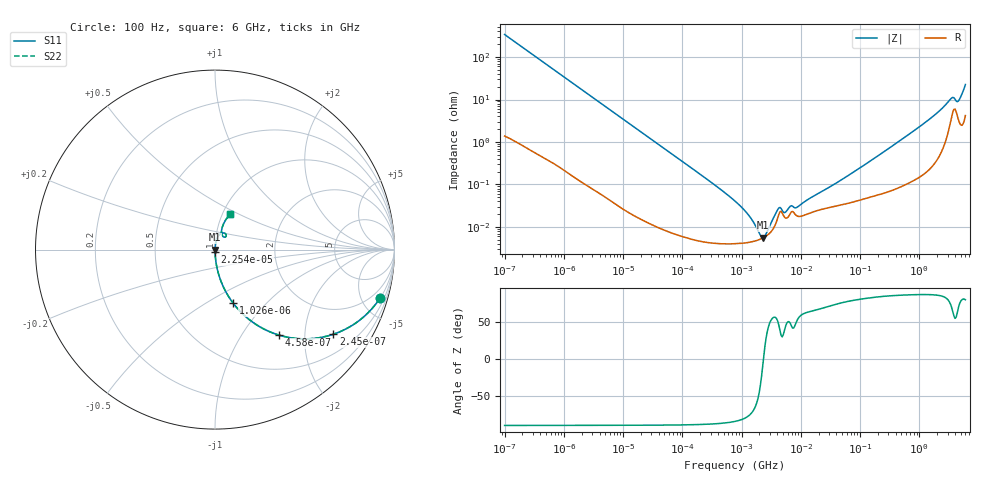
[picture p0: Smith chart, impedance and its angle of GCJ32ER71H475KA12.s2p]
!Murata Part Number: GCJ32ER71H475KA12
!These Parameters are Measured in Series Mode Connection
!Data Generated on Mar 13, 2026
!  o--ll--o
!Port1  Port2
!  o------o
!Operation Temp=25[degC], DC Bias Voltage=0[V]
!Freq. Start=100[Hz] Stop=6[GHz] 401[Steps]
# Hz S RI R 50
!Freq.(Hz) S11(Real) S11(Imag) S21(Real) S21(Imag) S12(Real) S12(Imag) S22(Real) S22(Imag)
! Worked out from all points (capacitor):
!   401 points, 100 Hz to 6 GHz, reference 50 ohm
!   read as one part in series: C = 4.68 uF near 109 Hz
!   lowest |Z| = 5.56 mohm at 2.269 MHz (marker M1)
!   series resonance near 2.344 MHz, so ESL is about 990 pH
!   S11 on the Smith chart (normalised r, x): 100 Hz: 1.03, -6.80; 245 Hz: 1.01, -2.78; 458 Hz: 1.01, -1.49; 1.026 kHz: 1.00, -0.67; 22.54 kHz: 1.00, -0.03; 6 GHz: 1.08, +0.44
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100  0.9194 -0.2702  0.0806 0.2702  0.0806 0.2702  0.9194 -0.2702
245  0.6588 -0.4716  0.3412 0.4716  0.3412 0.4716  0.6588 -0.4716
458  0.3578 -0.4765  0.6422 0.4765  0.6422 0.4765  0.3578 -0.4765
1026  0.1019 -0.2993  0.8981 0.2993  0.8981 0.2993  0.1019 -0.2993
2008  0.0295 -0.1659  0.9705 0.1659  0.9705 0.1659  0.0295 -0.1659
22537  0.000376 -0.0154  0.9996 0.0154  0.9996 0.0154  0.000376 -0.0154
40335  0.000169 -0.00862  0.9998 0.00862  0.9998 0.00862  0.000169 -0.00862
774597  4.04e-05 -0.000405  1 0.000405  1 0.000405  4.04e-05 -0.000405
1212075  4.26e-05 -0.000214  1 0.000214  1 0.000214  4.26e-05 -0.000214
1734173  4.73e-05 -9.35e-05  1 9.35e-05  1 9.35e-05  4.73e-05 -9.35e-05
2268635  5.47e-05 -1.01e-05  0.9999 1.01e-05  0.9999 1.01e-05  5.47e-05 -1.01e-05
2967816  7.09e-05 7.75e-05  0.9999 -7.75e-05  0.9999 -7.75e-05  7.09e-05 7.75e-05
4246196  0.000196 0.000199  0.9998 -0.000199  0.9998 -0.000199  0.000196 0.000199
5554849  0.000162 0.000157  0.9998 -0.000157  0.9998 -0.000157  0.000162 0.000157
6644369  0.000208 0.000227  0.9998 -0.000227  0.9998 -0.000227  0.000208 0.000227
8692127  0.000181 0.00023  0.9998 -0.00023  0.9998 -0.00023  0.000181 0.00023
1.555665e7  0.000222 0.00046  0.9998 -0.00046  0.9998 -0.00046  0.000222 0.00046
3.124326e8  0.000738 0.00719  0.9993 -0.00719  0.9993 -0.00719  0.000738 0.00719
1.497423e9  0.00349 0.0345  0.9965 -0.0345  0.9965 -0.0345  0.00349 0.0345
3.352442e9  0.0365 0.0913  0.9635 -0.0913  0.9635 -0.0913  0.0365 0.0913
4.586474e9  0.039 0.0806  0.961 -0.0806  0.961 -0.0806  0.039 0.0806
6e9  0.0819 0.1956  0.9181 -0.1956  0.9181 -0.1956  0.0819 0.1956
